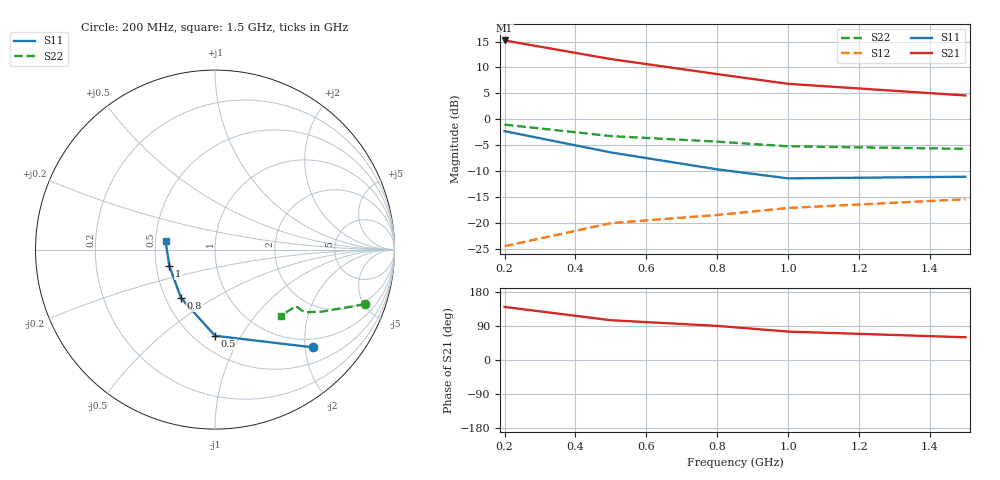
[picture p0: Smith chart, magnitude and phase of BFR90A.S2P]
!  BFR90A.S2P
!  BFR90
!  VCE=5V; IC=2mA
#  GHZ S MA R 50
!  S-PARAMETER DATA
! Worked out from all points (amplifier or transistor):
!   5 points, 200 MHz to 1.5 GHz, reference 50 ohm
!   highest |S21| = 15.2 dB at 200 MHz (marker M1)
!   |S21| within 3 dB of that: start of sweep to 450.7 MHz
!   unconditionally stable (mu >= 1): 907.9 MHz to end of sweep
!   at 200 MHz: K = 0.30, MSG = 19.8 dB, |S12| = -24.4 dB
!   at 800 MHz: K = 0.90, MSG = 13.6 dB, |S12| = -18.4 dB
!   at 1.5 GHz: K = 1.16, MAG = 7.5 dB, |S12| = -15.4 dB
!   S11 on the Smith chart (normalised r, x): 200 MHz: 0.81, -2.16; 500 MHz: 0.63, -0.78; 800 MHz: 0.60, -0.36; 1 GHz: 0.59, -0.12; 1.5 GHz: 0.57, +0.06
0.2  0.77 -45.0  5.76 140.0  0.06 65.0  0.89 -20.0
0.5  0.48 -90.0  3.81 105.0  0.1 55.0  0.69 -30.0
0.8  0.33 -125.0  2.73 90.0  0.12 55.0  0.61 -35.0
1  0.27 -160.0  2.2 75.0  0.14 55.0  0.55 -35.0
1.5  0.28 170.0  1.7 60.0  0.17 55.0  0.52 -45.0
